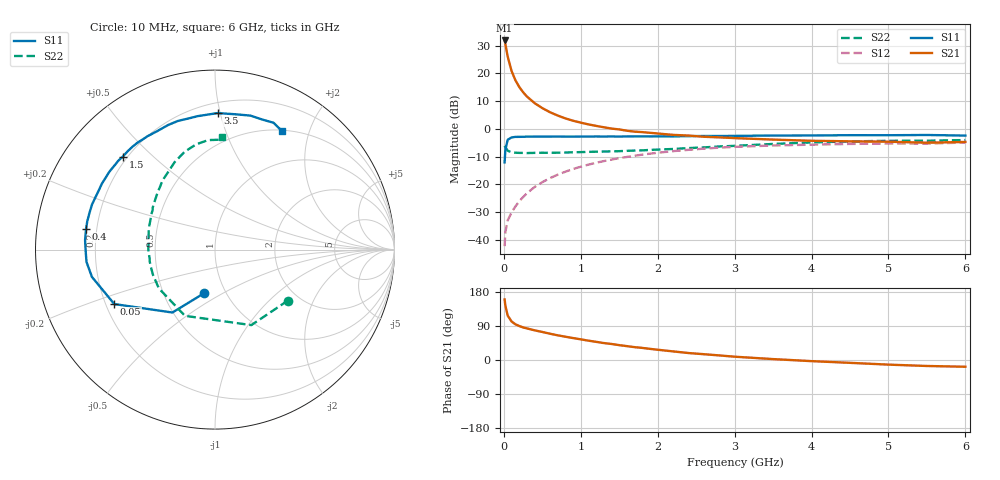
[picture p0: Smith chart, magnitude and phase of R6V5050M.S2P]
! SIEMENS Small Signal Semiconductors
! BFR193
! Si NPN RF Bipolar Junction Transistor in SOT23
! VCE = 0.5 V  IC = 50 mA
! Common Emitter S-Parameters:  May  1996
# GHz  S  MA  R  50
!  f  S11  S21  S12  S22
! GHz  MAG  ANG  MAG  ANG  MAG  ANG  MAG  ANG
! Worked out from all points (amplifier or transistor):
!   36 points, 10 MHz to 6 GHz, reference 50 ohm
!   highest |S21| = 31.9 dB at 10 MHz (marker M1)
!   |S21| within 3 dB of that: start of sweep to 31.18 MHz
!   unconditionally stable (mu >= 1): start of sweep to 13.51 MHz; 150 MHz to end of sweep
!   at 250 MHz: K = 1.11, MAG = 16.9 dB, |S12| = -24.6 dB
!   at 1.4 GHz: K = 1.10, MAG = 3.6 dB, |S12| = -11.0 dB
!   at 6 GHz: K = 1.03, MAG = -0.9 dB, |S12| = -4.9 dB
!   S11 on the Smith chart (normalised r, x): 10 MHz: 0.79, -0.41; 50 MHz: 0.23, -0.24; 400 MHz: 0.16, +0.08; 1.5 GHz: 0.18, +0.41; 3.5 GHz: 0.27, +0.98; 6 GHz: 0.51, +1.59
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0.01  0.2496 -103.8  39.41 159.7  0.0077 67.2  0.4957 -34.9
0.02  0.4234 -124.1  33.8 143.4  0.0139 58.3  0.4669 -64.3
0.05  0.6379 -151.6  20.2 117.3  0.0224 51.9  0.4052 -114.4
0.1  0.7024 -167.5  11.13 101.7  0.0311 56.6  0.38 -145.3
0.15  0.7192 -174.5  7.567 94.3  0.04 60.6  0.3732 -157.8
0.2  0.7201 -178.7  5.727 89.7  0.0495 64.6  0.3702 -164.8
0.25  0.7226 178.2  4.603 86.0  0.0592 66.2  0.3698 -169.5
0.3  0.7258 175.8  3.844 83.4  0.0694 67.7  0.3676 -172.7
0.4  0.7277 170.9  2.921 78.3  0.0897 68.6  0.3706 -177.8
0.5  0.7289 167.5  2.375 74.0  0.1098 68.1  0.3719 178.2
0.6  0.7286 163.6  2.003 69.4  0.1298 67.1  0.3713 175.1
0.7  0.7299 159.8  1.745 65.1  0.1497 66.0  0.3731 172.6
0.9  0.7267 153.1  1.406 57.9  0.1897 62.7  0.3794 167.1
1.1  0.7291 146.9  1.208 51.0  0.2273 59.2  0.3861 162.8
1.5  0.7295 134.7  0.981 39.2  0.2973 51.3  0.3974 154.4
1.7  0.7348 128.7  0.894 33.9  0.3285 47.3  0.4081 149.5
2.2  0.7344 116.0  0.782 22.7  0.3979 37.4  0.4356 139.6
3  0.7497 97.5  0.684 8.7  0.4755 22.5  0.4957 123.5
3.5  0.7608 88.9  0.643 2.4  0.5034 14.2  0.5365 114.8
4.5  0.7722 75.2  0.598 -7.5  0.5366 1.1  0.5959 100.1
5.5  0.7784 65.2  0.565 -15.8  0.5442 -10.4  0.614 86.2
6  0.759 60.7  0.583 -17.8  0.5688 -14.1  0.6306 86.7
